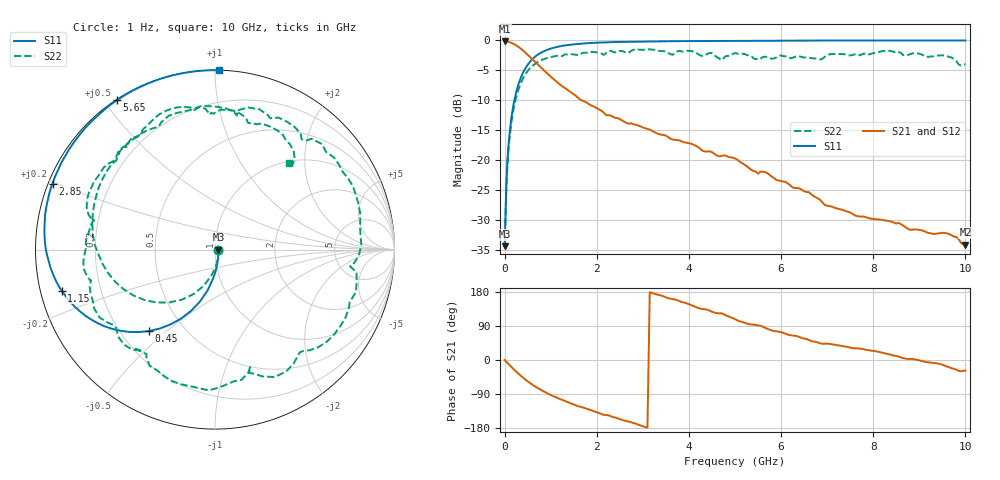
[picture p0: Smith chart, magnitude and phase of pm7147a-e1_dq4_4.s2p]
# GHz S DB R 50
! S-Parameters data
! Freq  dbS11  angS11  dbS21  angS21  dbS12  angS12  dbS22  angS22
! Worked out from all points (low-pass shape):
!   279 points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, 1 Hz to 10 GHz, reference 50 ohm
!   highest |S21| = -0.17 dB at 631 Hz (marker M1); lowest = -34.1 dB at 10 GHz (marker M2)
!   |S21| within 3 dB of the highest: start of sweep to 605.4 MHz
!   lowest |S11| = -34.4 dB at 1 kHz (marker M3), VSWR 1.04, Z = 51.9 - j0.00016 ohm
!   |S11| at or under -10 dB: start of sweep to 211.9 MHz
!   |S22| runs from -34.4 to -1.5 dB; largest |S21 - S12| = 5.2e-14
!   S11 on the Smith chart (normalised r, x): 1 Hz: 1.04, -0.00; 450 MHz: 0.32, -0.44; 1.15 GHz: 0.06, -0.13; 2.85 GHz: 0.01, +0.20; 5.65 GHz: 0.00, +0.54; 10 GHz: 0.00, +1.02
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1e-09  -34.37 -0.0  -0.17 -0.0  -0.17 -0.0  -34.37 -0.0
6.31e-07  -34.37 -0.0  -0.17 -0.0  -0.17 -0.0  -34.37 -0.0
1e-06  -34.37 -0.0  -0.17 -0.0  -0.17 -0.0  -34.37 -0.0
0.06309573  -19.94 -85.3  -0.21 -8.0  -0.21 -8.0  -20.69 -87.4
0.15  -12.73 -100.3  -0.41 -18.7  -0.41 -18.7  -13.51 -107.3
0.45  -4.67 -129.0  -2.03 -51.6  -2.03 -51.6  -5.66 -150.6
0.75  -2.22 -148.2  -4.25 -76.2  -4.25 -76.2  -3.47 177.7
1.15  -1.06 -165.0  -7.00 -100.4  -7.00 -100.4  -2.56 144.2
1.7  -0.50 179.5  -10.08 -125.1  -10.08 -125.1  -2.05 109.0
2.25  -0.29 168.1  -12.47 -146.0  -12.47 -146.0  -1.80 76.9
2.85  -0.20 157.9  -14.07 -167.8  -14.07 -167.8  -1.68 41.4
3.35  -0.15 150.6  -15.65 171.5  -15.65 171.5  -1.76 8.1
3.8  -0.12 144.5  -16.71 155.3  -16.71 155.3  -1.73 -16.8
4.15  -0.10 140.0  -17.61 139.9  -17.61 139.9  -2.03 -43.4
5.05  -0.06 129.6  -19.91 104.5  -19.91 104.5  -2.20 -97.2
5.65  -0.04 123.2  -21.99 85.5  -21.99 85.5  -2.71 -133.6
6.1  -0.03 118.7  -23.65 69.3  -23.65 69.3  -2.65 -159.9
6.7  -0.02 113.1  -25.97 49.0  -25.97 49.0  -3.00 171.1
7.2  -0.01 108.8  -28.04 39.3  -28.04 39.3  -2.23 150.3
8.35  -0.01 99.6  -30.19 14.8  -30.19 14.8  -1.73 104.6
9.75  -0.00 90.1  -32.78 -23.2  -32.78 -23.2  -3.10 51.2
10  -0.00 88.6  -34.10 -27.9  -34.10 -27.9  -3.98 49.4
